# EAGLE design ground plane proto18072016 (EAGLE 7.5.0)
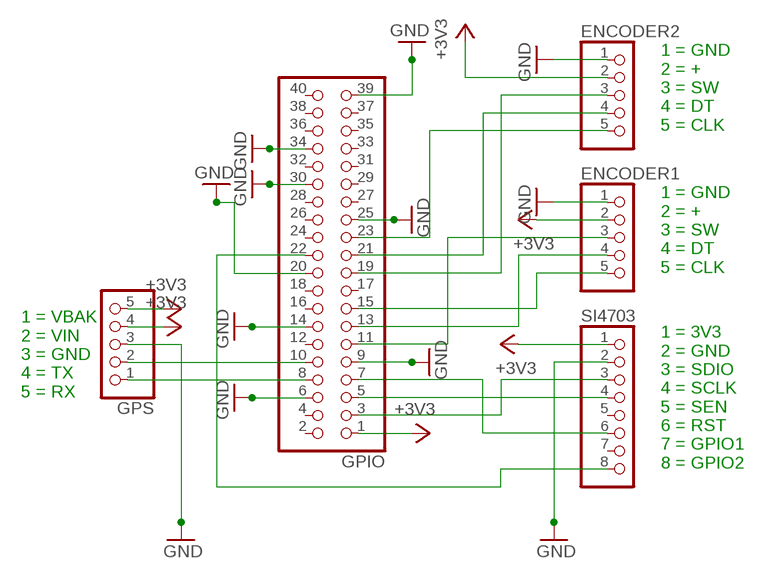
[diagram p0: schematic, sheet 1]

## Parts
ENCODER1  PINHD-1X5  [1X05]
ENCODER2  PINHD-1X5  [1X05]
GPIO  PINHD-2X20  [2X20]
GPS  PINHD-1X5  [1X05]
SI4703  PINHD-1X8  [1X08]

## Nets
+3V3: ENCODER1.2 ENCODER2.2 GPIO.1 GPS.4 GPS.5 SI4703.1
GND: ENCODER1.1 ENCODER2.1 GPIO.6 GPIO.9 GPIO.14 GPIO.20 GPIO.25 GPIO.30 GPIO.34 GPIO.39 GPS.3 SI4703.2
N$1: ENCODER1.3 GPIO.11
N$2: ENCODER1.4 GPIO.13
N$3: ENCODER1.5 GPIO.15
N$4: GPIO.3 SI4703.3
N$5: GPIO.5 SI4703.4
N$6: GPIO.7 SI4703.6
N$8: ENCODER2.3 GPIO.19
N$9: ENCODER2.4 GPIO.21
N$10: ENCODER2.5 GPIO.23
N$11: GPIO.8 GPS.1
N$12: GPIO.10 GPS.2
N$15: GPIO.22 SI4703.8
Unconnected: GPIO.2 GPIO.4 GPIO.12 GPIO.16 GPIO.17 GPIO.18 GPIO.24 GPIO.26 GPIO.27 GPIO.28 GPIO.29 GPIO.31 GPIO.32 GPIO.33 GPIO.35 GPIO.36 GPIO.37 GPIO.38 GPIO.40 SI4703.5 SI4703.7

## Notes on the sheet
- 1 = GND
  2 = +
  3 = SW
  4 = DT
  5 = CLK
- 1 = GND
  2 = +
  3 = SW
  4 = DT
  5 = CLK
- 1 = VBAK
  2 = VIN
  3 = GND
  4 = TX
  5 = RX
- 1 = 3V3
  2 = GND
  3 = SDIO
  4 = SCLK
  5 = SEN
  6 = RST
  7 = GPIO1
  8 = GPIO2

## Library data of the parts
ENCODER1 ENCODER2 GPS = pinhead:PINHD-1X5: PIN HEADER
GPIO = pinhead:PINHD-2X20: PIN HEADER
SI4703 = pinhead:PINHD-1X8: PIN HEADER

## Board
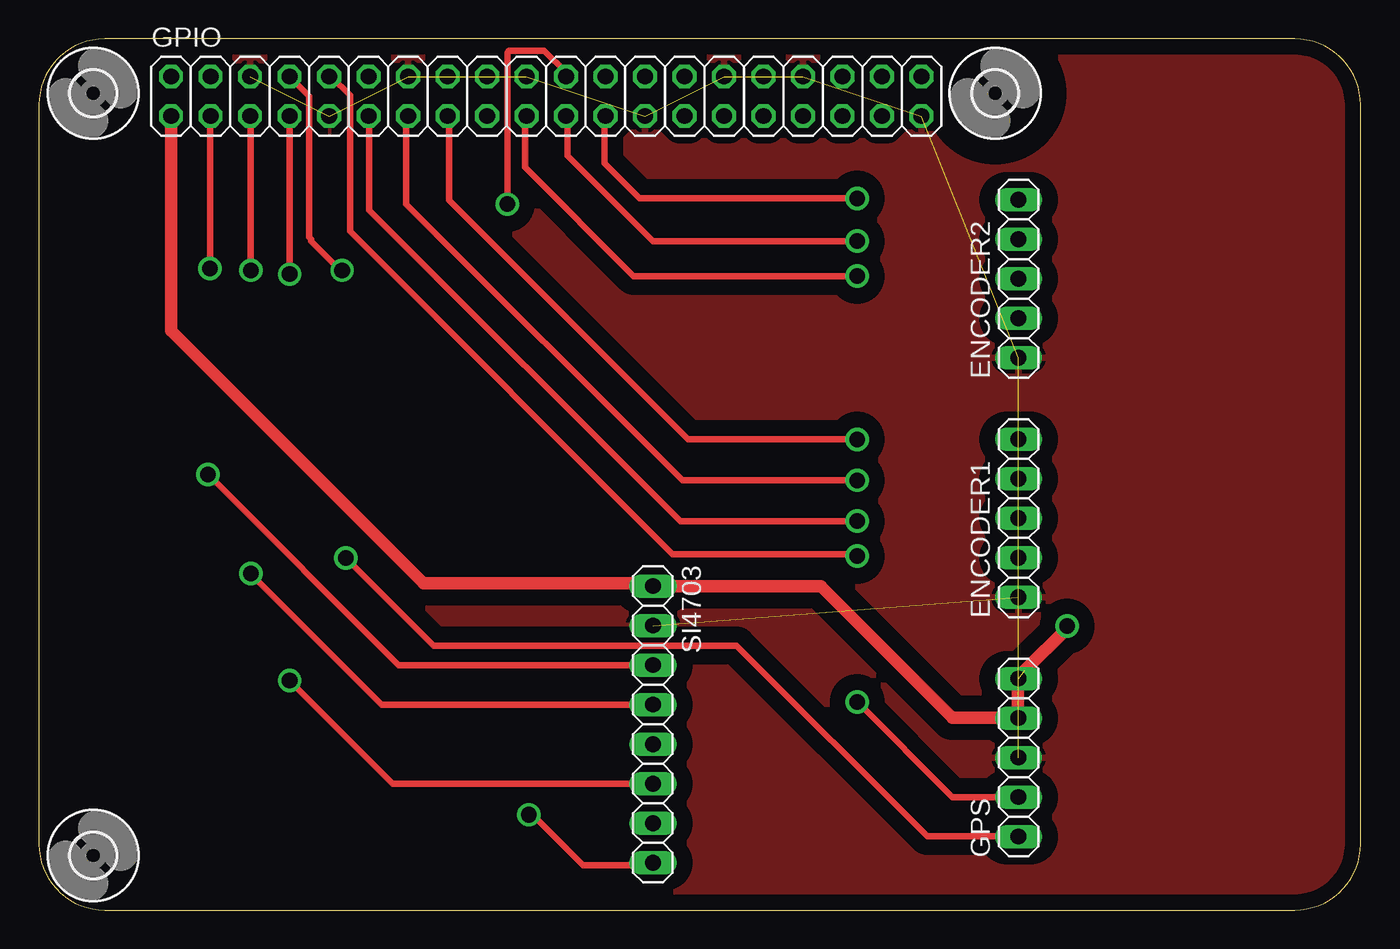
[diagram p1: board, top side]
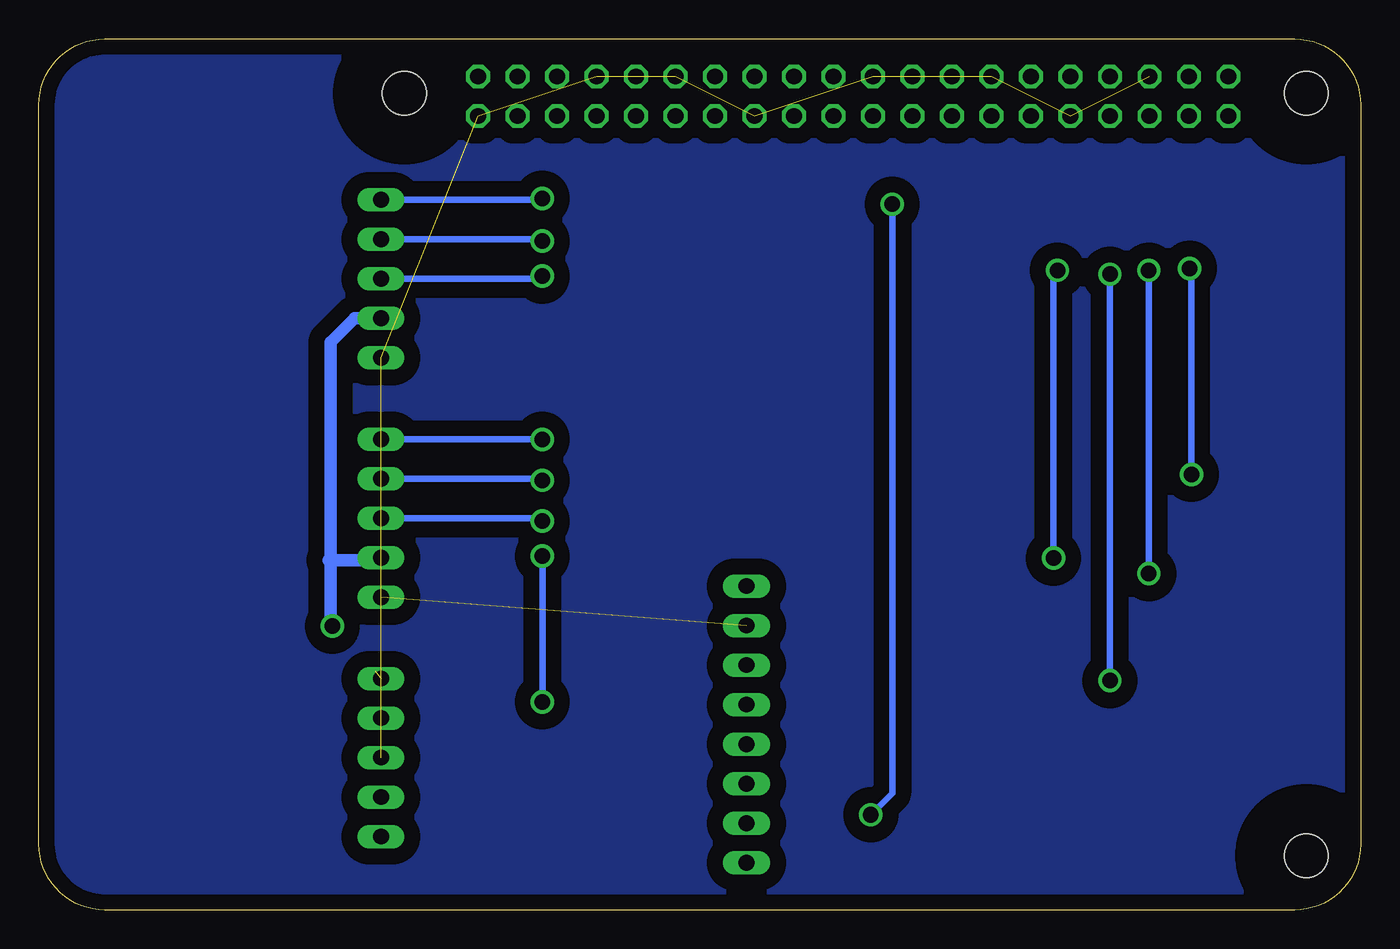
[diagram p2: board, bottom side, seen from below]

Size 85 x 56 mm. Coordinates in mm from the lower left corner, seen from the top.
Outline: 0,51.76 0,4.24 arc90 4.24,0 80.76,0 arc90 85,4.24 85,51.76 arc90 80.76,56 4.24,56 arc90 0,51.76
Copper layers (1*16): Top 0.035mm / dielectric 1.5mm / Bottom 0.035mm
Design rules "default": minimum track width 10mil, minimum drill 24mil, track to track 8mil, track to pad 8mil, pad to pad 8mil, via to via 8mil, smd to smd 8mil, copper to edge 40mil, drill to drill 8mil, minimum pad ring 10mil, minimum via ring 8mil, stop-mask expansion 4mil, vias tented up to drill 0mil, thermal gap 10mil

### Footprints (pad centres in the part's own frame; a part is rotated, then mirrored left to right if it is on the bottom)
1X05 = drill 1.016 long: 1 -5.08,0; 2 -2.54,0; 3 0,0; 4 2.54,0; 5 5.08,0
2X20 = drill 1.016 octagon: 1 -24.13,-1.27; 2 -24.13,1.27; 3 -21.59,-1.27; 4 -21.59,1.27; 5 -19.05,-1.27; 6 -19.05,1.27; 7 -16.51,-1.27; 8 -16.51,1.27; 9 -13.97,-1.27; 10 -13.97,1.27; 11 -11.43,-1.27; 12 -11.43,1.27; 13 -8.89,-1.27; 14 -8.89,1.27; 15 -6.35,-1.27; 16 -6.35,1.27; 17 -3.81,-1.27; 18 -3.81,1.27; 19 -1.27,-1.27; 20 -1.27,1.27; 21 1.27,-1.27; 22 1.27,1.27; 23 3.81,-1.27; 24 3.81,1.27; 25 6.35,-1.27; 26 6.35,1.27; 27 8.89,-1.27; 28 8.89,1.27; 29 11.43,-1.27; 30 11.43,1.27; 31 13.97,-1.27; 32 13.97,1.27; 33 16.51,-1.27; 34 16.51,1.27; 35 19.05,-1.27; 36 19.05,1.27; 37 21.59,-1.27; 38 21.59,1.27; 39 24.13,-1.27; 40 24.13,1.27
1X08 = drill 1.016 long: 1 -8.89,0; 2 -6.35,0; 3 -3.81,0; 4 -1.27,0; 5 1.27,0; 6 3.81,0; 7 6.35,0; 8 8.89,0
2,8 = hole 2.8: 0,0

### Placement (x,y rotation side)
ENCODER1  63,25.18 90 top
ENCODER2  63,40.58 90 top
GPIO  32.63,52.31 0 top
GPS  63,9.8 90 top
SI4703  39.49,11.94 270 top
U$1  [2,8]  3.5,3.5 0 top
U$2  [2,8]  3.5,52.5 0 top
U$3  [2,8]  61.5,52.5 0 top

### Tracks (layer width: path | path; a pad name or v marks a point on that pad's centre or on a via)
+3V3  (via drill 1)  (2 unrouted)
  Top 0.813: GPIO.1 8.5,37.25 24.75,21 39.31,21 SI4703.1 50.3,20.82 58.75,12.38 62.97,12.38 | 62.97,12.38 GPS.4 | 62.97,12.38 62.97,14.85 GPS.5 | v66.12,18.25 66.12,18.12 63.38,15.38
  Bottom 0.813: ENCODER2.2 64.71,38.04 66.25,36.5 66.25,18.38 v66.12,18.25
GND  (11 unrouted)
  pour Top (isolate 1.016): 6.7,55.9 arc-90 6.9,56.1 81.7,56.1 arc-90 85.2,52.6 85.2,48.9 85.2,5.3 arc-90 79.9,0 79,0 6.6,0 arc-90 0.1,6.5 0.1,7 0.1,48.7 arc-90 7.1,55.7 7.4,55.7
N$1  (via drill 1)
  Top 0.406: v52.62,25 41.25,25 21.25,45 21.25,50.99 GPIO.11
  Bottom 0.406: ENCODER1.3 52.81,25.18 v52.62,25
N$2  (via drill 1)
  Top 0.406: v52.62,27.62 41.38,27.62 23.62,45.38 23.62,50.92 GPIO.13
  Bottom 0.406: ENCODER1.4 52.73,27.73 v52.62,27.62
N$3  (via drill 1)
  Top 0.406: v52.62,30.25 41.75,30.25 26.38,45.62 26.38,50.95 GPIO.15
  Bottom 0.406: ENCODER1.5 52.64,30.27 v52.62,30.25
N$4  (via drill 1)
  Top 0.406: SI4703.3 23.13,15.74 v10.88,28 | v11,41.25 11,51 GPIO.3
  Bottom 0.406: v10.88,28 10.88,41.12 v11,41.25
N$5  (via drill 1)
  Top 0.406: SI4703.4 22.05,13.21 v13.62,21.62 | v13.62,41.12 13.62,50.99 GPIO.5
  Bottom 0.406: v13.62,21.62 v13.62,41.12
N$6  (via drill 1)
  Top 0.406: SI4703.6 22.75,8.12 v16.12,14.75 | v16.12,40.88 GPIO.7
  Bottom 0.406: v16.12,14.75 v16.12,40.88
N$7
  Bottom 0.813: 63.25,22.5 66.38,22.5
N$8  (via drill 1)
  Top 0.406: v52.62,40.75 38.25,40.75 31.25,47.75 31.25,50.93 GPIO.19
  Bottom 0.406: ENCODER2.3 52.8,40.58 v52.62,40.75
N$9  (via drill 1)
  Top 0.406: v52.62,43 39.5,43 34,48.5 34,50.94 GPIO.21
  Bottom 0.406: ENCODER2.4 52.74,43.12 v52.62,43
N$10  (via drill 1)
  Top 0.406: v52.62,45.75 38.62,45.75 36.38,48 36.38,50.98 GPIO.23
  Bottom 0.406: ENCODER2.5 52.72,45.66 v52.62,45.75
N$11  (via drill 1)
  Top 0.406: GPS.1 63,4.75 57.12,4.75 44.88,17 25.38,17 v19.75,22.62 | v19.5,41.12 19.38,41.12 17.5,43 17.5,43.12 17.38,43.25 17.38,52.33 GPIO.8
  Bottom 0.406: v19.75,22.62 19.75,40.88 v19.5,41.12
N$12  (via drill 1)
  Top 0.406: GPS.2 58.74,7.26 v52.62,13.38 | GPIO.10 18.8,53.58 20,52.38 20,43.62 40.75,22.88 52.62,22.88 | 52.62,22.88 53,22.88 53.12,22.75 | v52.62,22.75 52.62,22.88
  Bottom 0.406: v52.62,13.38 v52.62,22.75 52.62,22.88
N$13
  pour Bottom (isolate 1.016): 7.5,56 78.7,56 arc-90 85.3,49.4 85.3,48.2 arc90 85.2,48.1 85.2,5.7 arc-90 79.6,0.1 75.2,0.1 6.1,0.1 arc-90 0.1,6.1 0.1,8.9 arc-90 -0.1,9.1 -0.1,51.9 arc-90 4.1,56.1 8.8,56.1
N$15  (via drill 1)
  Top 0.406: GPIO.22 33.9,53.85 32.5,55.25 30.25,55.25 30.12,55.12 v30.12,45.38 | v31.5,6.12 31.75,6.12 35,2.88 39.32,2.88 SI4703.8
  Bottom 0.406: v30.12,45.38 30.12,7.5 v31.5,6.12 31.88,5.75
